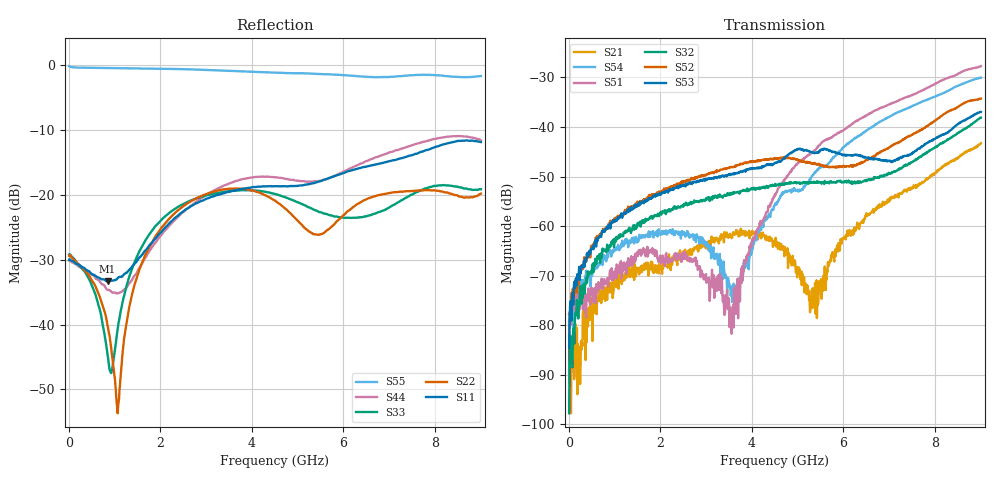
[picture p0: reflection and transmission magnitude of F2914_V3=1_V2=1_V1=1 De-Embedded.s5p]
! Integrated Device Technology
! Corporate Headquarters
! 6024 Silver Creek Valley Road
! San Jose, CA 95138  USA
! Phone:  1-408-284-8200
! Toll Free:  1-800-223-1366
! Webpage:  http://www.idt.com/
! Timing and RF Division
! 515 Groton Road, Suite 102
! Westford, MA 01886-6024
! Device:  F2914
! Description: High Reliability SP4T RF Switch
! Frequency:  0.05 -  8.GHz
! Package:  4x4 mm Thin QFN Plastic Package: 24 pin
! Ports:  5 RF,  5 DC
!  Pin  1  = GND
!  Pin  2  = GND
!  Pin  3  = GND
!  Pin  4  = GND
!  Pin  5  = RF4  =  Port 4
!  Pin  6  = GND
!  Pin  7  = GND
!  Pin  8  = RF3  =  Port 3
!  Pin  9  = GND
!  Pin 10  = GND
!  Pin 11  = RF2  =  Port 2
!  Pin 12  = GND
!  Pin 13  = GND
!  Pin 14  = RF1  =  Port 1
!  Pin 15  = GND
!  Pin 16  = Vcc
!  Pin 17  = V1
!  Pin 18  = V2
!  Pin 19  = V3
!  Pin 20  = VSSext
!  Pin 21  = GND
!  Pin 22  = RFC  =  Port 5
!  Pin 23  = GND
!  Pin 24  = GND
! Voltage:  VDD  =  +3.30 Volts
!  VSSEXT =  0.00 Volts
! Current:  IDD  = 336  uA
! State:  All OFF
! V1:  Logic HIGH
! V2:  Logic HIGH
! V3:  Logic HIGH
! Data:  The device was measured on the F291x evaluation board which has
!  individual transmission lines to the RF pins.  Data was collected
!  using a calibrated network analyzer.  The input lines were
!  modeled using Automatic Fixture Removal (AFR) from Keysight.
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# Hz S  dB  R 50
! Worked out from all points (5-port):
!   900 points, 10 MHz to 9 GHz, reference 50 ohm
!   strongest paths, dB at 10 MHz, 2.26 GHz, 4.51 GHz, 6.76 GHz, 9 GHz:
!     S53: -84.6, -52.7, -47.3, -46.5, -37.0
!     S52: -77.7, -52.1, -46.4, -45.3, -34.3
!     S32: -97.8, -56.6, -51.5, -50.1, -38.1
!     S51: -81.5, -67.2, -53.8, -36.4, -27.7
!     S54: -82.5, -61.6, -55.6, -39.1, -30.0
!     S21: -79.3, -67.8, -63.1, -55.9, -43.3
!   lowest |S11| = -33.3 dB at 850 MHz (marker M1), VSWR 1.04, Z = 48.6 + j1.59 ohm
!   |S11| at or under -10 dB: start of sweep to end of sweep
